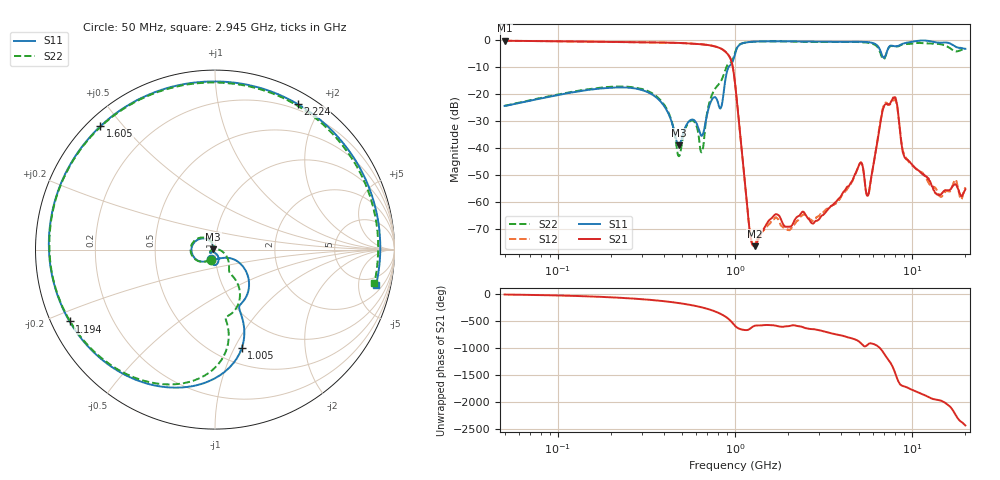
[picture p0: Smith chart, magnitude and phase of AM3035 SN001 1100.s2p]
# Hz S DB R 50
!freq MagS11 AngS11 MagS21 AngS21 MagS12 AngS12 MagS22 AngS22
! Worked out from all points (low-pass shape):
!   1601 points, 50 MHz to 20.05 GHz, reference 50 ohm
!   highest |S21| = -0.37 dB at 50 MHz (marker M1); lowest = -76.4 dB at 1.292 GHz (marker M2)
!   |S21| within 3 dB of the highest: start of sweep to 839.1 MHz
!   lowest |S11| = -39.1 dB at 482.3 MHz (marker M3), VSWR 1.02, Z = 48.9 + j0.071 ohm
!   |S11| at or under -10 dB: start of sweep to 923.3 MHz
!   |S22| runs from -43.1 to -0.6 dB; largest |S21 - S12| = 0.011
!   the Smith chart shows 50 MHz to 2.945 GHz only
!   S11 on the Smith chart (normalised r, x): 50 MHz: 0.95, -0.10; 1.005 GHz: 0.66, -1.07; 1.194 GHz: 0.05, -0.23; 1.605 GHz: 0.04, +0.44; 2.224 GHz: 0.14, +1.71; 2.945 GHz: 3.16, -8.00
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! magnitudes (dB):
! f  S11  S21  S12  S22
! 50 MHz  -24.5  -0.4  -0.4  -24.4
! 135.9 MHz  -18.9  -0.7  -0.7  -18.7
! 369.6 MHz  -22.0  -1.0  -1.0  -21.6
! 482.3 MHz  -39.1  -1.2  -1.2  -43.1
! 566.6 MHz  -29.6  -1.4  -1.4  -29.9
! 650.8 MHz  -35.6  -1.7  -1.7  -41.6
! 733.7 MHz  -22.7  -2.1  -2.1  -21.2
! 833.3 MHz  -25.2  -3.3  -3.2  -15.4
! 1.005 GHz  -4.9  -16.9  -16.9  -4.5
! 1.194 GHz  -0.9  -66.9  -66.5  -0.9
! 1.292 GHz  -0.7  -76.4  -75.7  -0.7
! 1.605 GHz  -0.6  -66.1  -67.2  -0.6
! 2.224 GHz  -0.6  -65.8  -67.4  -0.7
! 2.722 GHz  -0.7  -68.0  -67.1  -0.8
! 2.945 GHz  -0.7  -66.8  -65.4  -0.8
! 5.089 GHz  -0.8  -45.7  -45.7  -0.9
! 5.652 GHz  -0.9  -57.6  -57.8  -1.1
! 7.402 GHz  -2.8  -23.9  -24.0  -2.9
! 8.098 GHz  -2.4  -21.7  -22.6  -2.6
! 9.233 GHz  -1.2  -44.0  -43.6  -1.6
! 13.58 GHz  -0.9  -56.8  -54.8  -1.5
! 20.05 GHz  -3.4  -55.3  -54.6  -3.6
